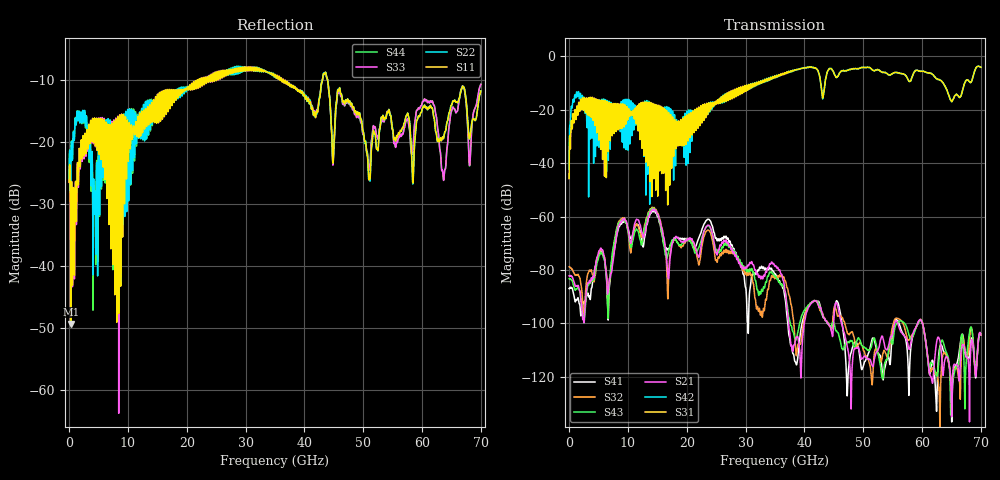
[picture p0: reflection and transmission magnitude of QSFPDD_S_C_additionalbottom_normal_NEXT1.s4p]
! AWR Design Environment (8415) Thu Dec 20 14:42:02 2018
! Document = 'CHANNEL TEST'
! nPorts: 4, nXvals: 7001
# HZ S DB R 50
!Freq DBS11 AngS11 DBS12 AngS12 DBS13 AngS13 DBS14 AngS14
!	DBS21 AngS21 DBS22 AngS22 DBS23 AngS23 DBS24 AngS24
!	DBS31 AngS31 DBS32 AngS32 DBS33 AngS33 DBS34 AngS34
!	DBS41 AngS41 DBS42 AngS42 DBS43 AngS43 DBS44 AngS44
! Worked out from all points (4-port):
!   7000 points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, 10 MHz to 70 GHz, reference 50 ohm
!   strongest paths, dB at 10 MHz, 17.51 GHz, 35.01 GHz, 52.51 GHz, 70 GHz:
!     S31: -45.8, -26.2, -7.4, -5.0, -4.0
!     S42: -42.2, -24.0, -7.5, -5.0, -4.0
!     S21: -82.2, -70.3, -78.6, -109.9, -104.3
!     S43: -83.3, -68.7, -82.4, -111.2, -104.2
!     S32: -78.8, -70.0, -83.1, -111.2, -104.2
!     S41: -87.0, -69.1, -81.5, -111.2, -104.3
!   lowest |S11| = -49.4 dB at 270 MHz (marker M1), VSWR 1.01, Z = 49.7 - j0.103 ohm
!   |S11| at or under -10 dB: start of sweep to 21.8 GHz; 36.46 GHz to 43.06 GHz (6.604 GHz wide, 16.6 % of centre); 43.96 GHz to end of sweep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
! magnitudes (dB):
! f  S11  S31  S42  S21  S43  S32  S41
! 10 MHz  -26.5  -45.8  -42.2  -82.2  -83.3  -78.8  -87.0
! 270 MHz  -49.4  -31.2  -22.7  -82.2  -83.4  -79.1  -86.5
! 14.21 GHz  -16.8  -17.8  -18.5  -57.4  -57.0  -56.8  -57.8
! 16.8 GHz  -14.1  -29.0  -30.3  -82.1  -74.1  -90.6  -72.0
! 23.63 GHz  -10.2  -18.9  -20.9  -63.2  -63.5  -65.0  -61.0
! 29.81 GHz  -8.2  -11.3  -11.9  -79.6  -79.6  -81.2  -83.3
! 70 GHz  -11.8  -4.0  -4.0  -104.3  -104.2  -104.2  -104.3
